| TEXAS INSTRUMENTS INCORPORATED
| Standard Linear and Logic Group
| IBIS Model of SN74CBT16212CC
| 24-Bit Fet Bus-exchange Switch with-2V Undershoot-Protection
| This file contains package information for the following:
|  SSOP 56-pin (DL) package as [Component] CBT16212C_DL
|  TSSOP 56-pin (DGG) package as [Component] CBT16212C_DGG
|  TVSOP 56-pin (DGV) package as [Component] CBT16212C_DGV
| This device can be powered at the following Vccs:
|  5 volt Vcc
|  4 volt Vcc
| This file provides unique models under the [Model Selector] for each Vcc.
| For operation at a specific Vcc, select the appropriate model after each
| [Model Selector] keyword.
[IBIS Ver]   3.2
[Comment char]  |_char
[File Name]   sn74cbt16212c.ibs
[File Rev]   1.1 | a_die
[Date]   July 28, 2003
[Source]   Data created from TI-SPICE simulations at TI-SLL.
[Notes]   The following is an IBIS list for the CBT16212C.
   Please contact sllibis@ti.com with questions and
   comments concerning SLL IBIS models.
   - Power clamp data deleted as there is no power-clamp diode.
   - Non-monotonic data due to FET characteristics.
[Disclaimer] Property of Texas Instruments Incorporated.  Unauthorized
   reproduction and/or distribution is strictly prohibited.
   This product is protected under copyright law.
   Created  2003, (C) Copyright  2003, Texas Instruments
   Incorporated, All Rights Reserved
   UNLESS THERE IS A SIGNED, WRITTEN AGREEMENT TO THE
   CONTRARY, TEXAS INSTRUMENTS (TI) IS PROVIDING THE IBIS
   MODELS  AND WITHOUT ANY WARRANTY, EXPRESSED OR
   IMPLIED.  TI assumes no liability for:
   1) the accuracy of the IBIS models provided to your
   company;
   2) the proper functioning of these IBIS Models in your
   design or for any resulting applications; or
   3) infringement of patents, copyrights or intellectual
   property rights resulting from your use of these IBIS
   models.
   TI provides IBIS Models as a service to our customers.
   You and your company shall not distribute, sell or give
   these models to anyone else without prior written
   permission from TI.
   TI reserves the right to make changes to our products or
   to discontinue any semiconductor product or service
   without notice, and advises our customers to obtain the
   latest version of relevant information to verify, before
   placing orders, that the information being relied on is
   current.
   Please be aware that your receipt and use of the IBIS
   information provided shall serve as acceptance of these
   terms and conditions.  If you do not accept these terms,
   you should return or destroy the IBIS models and any
   other accompanying information immediately.
| NOTE: GQL Component package is commented out below because different
| Series pin mapping.
| Component CBT16212C_DL 56-pin SSOP
[Component]   CBT16212C_DL
[Manufacturer]   Texas Instruments, Inc.
[Package]
|   typ   min   max
R_pkg   5.500e-02   4.800e-02   6.700e-02
L_pkg   6.539e-09   4.803e-09   9.746e-09
C_pkg   8.570e-13   5.000e-13   1.351e-12
[Pin]   signal_name   model_name   R_pin   L_pin   C_pin
1   S0   CBT16212C_CTRL   6.400e-02   9.646e-09   1.202e-12
2   1A1   CBT16212C_IO   5.900e-02   8.723e-09   1.348e-12
3   1A2   CBT16212C_IO   5.900e-02   8.139e-09   1.223e-12
4   2A1   CBT16212C_IO   5.600e-02   7.554e-09   1.088e-12
5   2A2   CBT16212C_IO   5.400e-02   6.991e-09   9.660e-13
6   3A1   CBT16212C_IO   5.300e-02   6.659e-09   9.730e-13
7   3A2   CBT16212C_IO   5.500e-02   6.321e-09   9.050e-13
8   GND   GND   5.600e-02   5.942e-09   7.130e-13
9   4A1   CBT16212C_IO   5.700e-02   5.768e-09   6.780e-13
10   4A2   CBT16212C_IO   5.400e-02   5.459e-09   6.310e-13
11   5A1   CBT16212C_IO   5.100e-02   5.224e-09   6.380e-13
12   5A2   CBT16212C_IO   4.800e-02   5.088e-09   6.010e-13
13   6A1   CBT16212C_IO   5.000e-02   5.021e-09   5.180e-13
14   6A2   CBT16212C_IO   5.100e-02   4.803e-09   5.000e-13
15   7A1   CBT16212C_IO   5.100e-02   4.803e-09   5.000e-13
16   7A2   CBT16212C_IO   5.000e-02   5.021e-09   5.180e-13
17   VCC   POWER   4.800e-02   5.088e-09   6.010e-13
18   8A1   CBT16212C_IO   5.100e-02   5.224e-09   6.380e-13
19   GND   GND   5.400e-02   5.459e-09   6.310e-13
20   8A2   CBT16212C_IO   5.700e-02   5.768e-09   6.770e-13
21   9A1   CBT16212C_IO   5.500e-02   5.942e-09   7.150e-13
22   9A2   CBT16212C_IO   5.500e-02   6.321e-09   9.070e-13
23   10A1   CBT16212C_IO   5.300e-02   6.659e-09   9.720e-13
24   10A2   CBT16212C_IO   5.400e-02   6.991e-09   9.660e-13
25   11A1   CBT16212C_IO   5.600e-02   7.554e-09   1.087e-12
26   11A2   CBT16212C_IO   5.900e-02   8.139e-09   1.223e-12
27   12A1   CBT16212C_IO   5.900e-02   8.727e-09   1.351e-12
28   12A2   CBT16212C_IO   6.700e-02   9.746e-09   1.210e-12
29   12B2   CBT16212C_IO   6.300e-02   9.630e-09   1.203e-12
30   12B1   CBT16212C_IO   6.000e-02   8.751e-09   1.349e-12
31   11B2   CBT16212C_IO   6.000e-02   8.184e-09   1.224e-12
32   11B1   CBT16212C_IO   5.600e-02   7.543e-09   1.087e-12
33   10B2   CBT16212C_IO   5.400e-02   7.005e-09   9.690e-13
34   10B1   CBT16212C_IO   5.600e-02   6.714e-09   9.750e-13
35   9B2   CBT16212C_IO   5.800e-02   6.384e-09   9.090e-13
36   9B1   CBT16212C_IO   5.700e-02   5.976e-09   7.170e-13
37   8B2   CBT16212C_IO   5.700e-02   5.743e-09   6.770e-13
38   GND   GND   5.400e-02   5.468e-09   6.310e-13
39   8B1   CBT16212C_IO   5.500e-02   5.329e-09   6.440e-13
40   7B2   CBT16212C_IO   5.200e-02   5.189e-09   6.060e-13
41   7B1   CBT16212C_IO   5.200e-02   5.053e-09   5.190e-13
42   6B2   CBT16212C_IO   5.200e-02   4.825e-09   5.020e-13
43   6B1   CBT16212C_IO   5.400e-02   4.897e-09   5.060e-13
44   5B2   CBT16212C_IO   5.200e-02   5.093e-09   5.210e-13
45   5B1   CBT16212C_IO   5.100e-02   5.179e-09   6.080e-13
46   4B2   CBT16212C_IO   5.400e-02   5.314e-09   6.450e-13
47   4B1   CBT16212C_IO   5.500e-02   5.511e-09   6.320e-13
48   3B2   CBT16212C_IO   5.700e-02   5.770e-09   6.770e-13
49   GND   GND   5.600e-02   5.956e-09   7.160e-13
50   3B1   CBT16212C_IO   5.500e-02   6.320e-09   9.050e-13
51   2B2   CBT16212C_IO   5.200e-02   6.621e-09   9.680e-13
52   2B1   CBT16212C_IO   5.300e-02   6.974e-09   9.660e-13
53   1B2   CBT16212C_IO   5.700e-02   7.571e-09   1.089e-12
54   1B1   CBT16212C_IO   5.700e-02   8.097e-09   1.219e-12
55   S2   CBT16212C_CTRL   5.900e-02   8.723e-09   1.349e-12
56   S1   CBT16212C_CTRL   6.100e-02   9.560e-09   1.199e-12
| Component CBT16212C_DGG 56-pin TSSOP
[Component]   CBT16212C_DGG
[Manufacturer]   Texas Instruments, Inc.
[Package]
|   typ   min   max
R_pkg   4.500e-02   3.500e-02   6.200e-02
L_pkg   3.324e-09   2.403e-09   5.094e-09
C_pkg   5.640e-13   3.410e-13   9.140e-13
[Pin]   signal_name   model_name   R_pin   L_pin   C_pin
1   S0   CBT16212C_CTRL   6.200e-02   5.094e-09   8.560e-13
2   1A1   CBT16212C_IO   6.100e-02   4.621e-09   9.020e-13
3   1A2   CBT16212C_IO   6.000e-02   4.316e-09   8.020e-13
4   2A1   CBT16212C_IO   5.900e-02   3.968e-09   6.980e-13
5   2A2   CBT16212C_IO   5.700e-02   3.716e-09   6.490e-13
6   3A1   CBT16212C_IO   4.200e-02   3.517e-09   6.530e-13
7   3A2   CBT16212C_IO   4.100e-02   3.160e-09   5.700e-13
8   GND   GND   3.900e-02   2.981e-09   4.820e-13
9   4A1   CBT16212C_IO   3.900e-02   2.808e-09   4.470e-13
10   4A2   CBT16212C_IO   3.800e-02   2.715e-09   4.090e-13
11   5A1   CBT16212C_IO   4.100e-02   2.675e-09   3.910e-13
12   5A2   CBT16212C_IO   3.900e-02   2.536e-09   3.660e-13
13   6A1   CBT16212C_IO   3.900e-02   2.457e-09   3.480e-13
14   6A2   CBT16212C_IO   3.800e-02   2.411e-09   3.530e-13
15   7A1   CBT16212C_IO   3.900e-02   2.456e-09   3.550e-13
16   7A2   CBT16212C_IO   3.900e-02   2.471e-09   3.490e-13
17   VCC   POWER   4.000e-02   2.580e-09   3.700e-13
18   8A1   CBT16212C_IO   3.800e-02   2.651e-09   3.890e-13
19   GND   GND   3.800e-02   2.739e-09   4.110e-13
20   8A2   CBT16212C_IO   3.900e-02   2.838e-09   4.490e-13
21   9A1   CBT16212C_IO   3.800e-02   2.988e-09   4.840e-13
22   9A2   CBT16212C_IO   3.800e-02   3.104e-09   5.640e-13
23   10A1   CBT16212C_IO   4.000e-02   3.427e-09   6.380e-13
24   10A2   CBT16212C_IO   5.600e-02   3.654e-09   6.410e-13
25   11A1   CBT16212C_IO   5.700e-02   3.932e-09   7.000e-13
26   11A2   CBT16212C_IO   5.800e-02   4.257e-09   8.060e-13
27   12A1   CBT16212C_IO   5.700e-02   4.580e-09   9.140e-13
28   12A2   CBT16212C_IO   5.900e-02   5.038e-09   8.610e-13
29   12B2   CBT16212C_IO   6.000e-02   5.058e-09   8.580e-13
30   12B1   CBT16212C_IO   5.600e-02   4.543e-09   9.040e-13
31   11B2   CBT16212C_IO   5.700e-02   4.241e-09   8.020e-13
32   11B1   CBT16212C_IO   5.900e-02   3.933e-09   6.990e-13
33   10B2   CBT16212C_IO   5.600e-02   3.616e-09   6.370e-13
34   10B1   CBT16212C_IO   3.700e-02   3.368e-09   6.400e-13
35   9B2   CBT16212C_IO   3.600e-02   3.024e-09   5.630e-13
36   9B1   CBT16212C_IO   3.500e-02   2.876e-09   4.740e-13
37   8B2   CBT16212C_IO   3.500e-02   2.745e-09   4.440e-13
38   GND   GND   3.700e-02   2.683e-09   4.050e-13
39   8B1   CBT16212C_IO   3.800e-02   2.603e-09   3.820e-13
40   7B2   CBT16212C_IO   3.800e-02   2.510e-09   3.620e-13
41   7B1   CBT16212C_IO   3.600e-02   2.412e-09   3.410e-13
42   6B2   CBT16212C_IO   3.800e-02   2.416e-09   3.490e-13
43   6B1   CBT16212C_IO   3.800e-02   2.403e-09   3.490e-13
44   5B2   CBT16212C_IO   3.700e-02   2.429e-09   3.410e-13
45   5B1   CBT16212C_IO   3.600e-02   2.483e-09   3.580e-13
46   4B2   CBT16212C_IO   3.700e-02   2.614e-09   3.810e-13
47   4B1   CBT16212C_IO   3.500e-02   2.669e-09   4.020e-13
48   3B2   CBT16212C_IO   3.600e-02   2.763e-09   4.420e-13
49   GND   GND   3.600e-02   2.942e-09   4.780e-13
50   3B1   CBT16212C_IO   3.500e-02   3.053e-09   5.640e-13
51   2B2   CBT16212C_IO   3.600e-02   3.408e-09   6.410e-13
52   2B1   CBT16212C_IO   5.800e-02   3.698e-09   6.410e-13
53   1B2   CBT16212C_IO   5.900e-02   3.974e-09   6.970e-13
54   1B1   CBT16212C_IO   6.100e-02   4.327e-09   8.020e-13
55   S2   CBT16212C_CTRL   6.100e-02   4.624e-09   9.050e-13
56   S1   CBT16212C_CTRL   6.000e-02   5.063e-09   8.580e-13
| Component CBT16212C_DGV 56-pin TVSOP
[Component]   CBT16212C_DGV
[Manufacturer]   Texas Instruments, Inc.
[Package]
|   typ   min   max
R_pkg   6.300e-02   5.000e-02   8.400e-02
L_pkg   2.945e-09   2.394e-09   3.939e-09
C_pkg   3.910e-13   2.710e-13   5.880e-13
[Pin]   signal_name   model_name   R_pin   L_pin   C_pin
1   S0   CBT16212C_CTRL   6.800e-02   3.933e-09   5.880e-13
2   1A1   CBT16212C_IO   6.800e-02   3.568e-09   5.870e-13
3   1A2   CBT16212C_IO   7.600e-02   3.464e-09   5.150e-13
4   2A1   CBT16212C_IO   8.400e-02   3.444e-09   4.590e-13
5   2A2   CBT16212C_IO   8.100e-02   3.277e-09   4.270e-13
6   3A1   CBT16212C_IO   7.400e-02   3.136e-09   3.870e-13
7   3A2   CBT16212C_IO   6.900e-02   2.970e-09   4.010e-13
8   GND   GND   5.000e-02   2.785e-09   3.790e-13
9   4A1   CBT16212C_IO   5.100e-02   2.685e-09   3.200e-13
10   4A2   CBT16212C_IO   5.300e-02   2.611e-09   3.160e-13
11   5A1   CBT16212C_IO   5.300e-02   2.495e-09   2.970e-13
12   5A2   CBT16212C_IO   5.300e-02   2.435e-09   2.920e-13
13   6A1   CBT16212C_IO   5.500e-02   2.412e-09   2.850e-13
14   6A2   CBT16212C_IO   5.600e-02   2.401e-09   2.730e-13
15   7A1   CBT16212C_IO   5.500e-02   2.401e-09   2.730e-13
16   7A2   CBT16212C_IO   5.500e-02   2.399e-09   2.840e-13
17   VCC   POWER   5.400e-02   2.406e-09   2.890e-13
18   8A1   CBT16212C_IO   5.300e-02   2.450e-09   2.930e-13
19   GND   GND   5.100e-02   2.544e-09   3.110e-13
20   8A2   CBT16212C_IO   5.100e-02   2.626e-09   3.150e-13
21   9A1   CBT16212C_IO   5.000e-02   2.727e-09   3.690e-13
22   9A2   CBT16212C_IO   6.500e-02   2.903e-09   3.930e-13
23   10A1   CBT16212C_IO   7.500e-02   3.091e-09   3.860e-13
24   10A2   CBT16212C_IO   8.200e-02   3.272e-09   4.280e-13
25   11A1   CBT16212C_IO   8.200e-02   3.393e-09   4.570e-13
26   11A2   CBT16212C_IO   7.300e-02   3.380e-09   5.080e-13
27   12A1   CBT16212C_IO   7.100e-02   3.577e-09   5.800e-13
28   12A2   CBT16212C_IO   6.800e-02   3.937e-09   5.740e-13
29   12B2   CBT16212C_IO   6.900e-02   3.923e-09   5.690e-13
30   12B1   CBT16212C_IO   6.400e-02   3.536e-09   5.740e-13
31   11B2   CBT16212C_IO   7.600e-02   3.428e-09   5.170e-13
32   11B1   CBT16212C_IO   8.100e-02   3.395e-09   4.680e-13
33   10B2   CBT16212C_IO   8.000e-02   3.255e-09   4.310e-13
34   10B1   CBT16212C_IO   7.100e-02   3.064e-09   3.860e-13
35   9B2   CBT16212C_IO   6.100e-02   2.878e-09   3.890e-13
36   9B1   CBT16212C_IO   5.000e-02   2.710e-09   3.630e-13
37   8B2   CBT16212C_IO   5.000e-02   2.606e-09   3.110e-13
38   GND   GND   5.200e-02   2.534e-09   3.060e-13
39   8B1   CBT16212C_IO   5.200e-02   2.439e-09   2.890e-13
40   7B2   CBT16212C_IO   5.300e-02   2.399e-09   2.860e-13
41   7B1   CBT16212C_IO   5.500e-02   2.394e-09   2.820e-13
42   6B2   CBT16212C_IO   5.500e-02   2.398e-09   2.710e-13
43   6B1   CBT16212C_IO   5.600e-02   2.396e-09   2.710e-13
44   5B2   CBT16212C_IO   5.400e-02   2.402e-09   2.830e-13
45   5B1   CBT16212C_IO   5.400e-02   2.423e-09   2.880e-13
46   4B2   CBT16212C_IO   5.300e-02   2.474e-09   2.920e-13
47   4B1   CBT16212C_IO   5.100e-02   2.569e-09   3.090e-13
48   3B2   CBT16212C_IO   5.100e-02   2.638e-09   3.130e-13
49   GND   GND   5.100e-02   2.742e-09   3.660e-13
50   3B1   CBT16212C_IO   6.400e-02   2.917e-09   3.900e-13
51   2B2   CBT16212C_IO   7.400e-02   3.083e-09   3.830e-13
52   2B1   CBT16212C_IO   8.100e-02   3.249e-09   4.300e-13
53   1B2   CBT16212C_IO   8.300e-02   3.400e-09   4.550e-13
54   1B1   CBT16212C_IO   7.500e-02   3.427e-09   5.050e-13
55   S2   CBT16212C_CTRL   7.100e-02   3.585e-09   5.780e-13
56   S1   CBT16212C_CTRL   6.900e-02   3.939e-09   5.810e-13
| Model CBT16212C_CTRL
[Model Selector]   CBT16212C_CTRL
CBT16212C_CTRL_50   5 volt Vcc
CBT16212C_CTRL_40   4 volt Vcc
| Model CBT16212C_IO
[Model Selector]   CBT16212C_IO
CBT16212C_IO_50   5 volt Vcc
CBT16212C_IO_40   4 volt Vcc
| Model CBT16212C_IO_S
[Model Selector]   CBT16212C_IO_S
CBT16212C_IO_50_S   5 volt Vcc_S
CBT16212C_IO_40_S   4 volt Vcc_S
[Model]   CBT16212C_IO_50_S
Model_type  Series_switch
| variable   typ   min   max
C_comp   0   0   0
[Temperature Range]   40   100   -40
| Ambient temperature   25   85   -40
[Voltage range]   5   4.5   5.5
[On]
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[Off]
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[Model]   CBT16212C_IO_40_S
Model_type  Series_switch
| variable   typ   min   max
C_comp   0   0   0
[Temperature Range]   40   100   -40
| Ambient temperature   25   85   -40
[Voltage range]   4   4   4
[On]
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[Off]
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| Models and submodels in the file (6): CBT16212C_CTRL_50 (Input), CBT16212C_CTRL_40 (Input), CBT16212C_IO_50_S (Series_switch), CBT16212C_IO_50 (Terminator), CBT16212C_IO_40_S (Series_switch), CBT16212C_IO_40 (Terminator)
